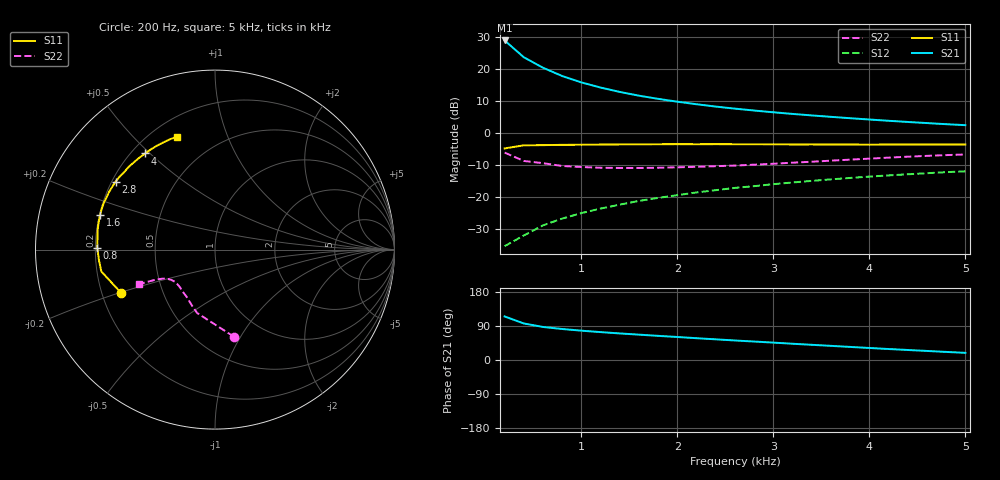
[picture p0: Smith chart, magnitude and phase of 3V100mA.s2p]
#  HZ  S  MA  R  50.0000
! Device:MCH4020
! Bias:VCE=3V, IC=100mA
!MHZ	S11(MAG/ANG)		S21(MAG/ANG)		S12(MAG/ANG)		S22(MAG/ANG)
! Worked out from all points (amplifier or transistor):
!   25 points, 200 Hz to 5 kHz, reference 50 ohm
!   highest |S21| = 29.0 dB at 200 Hz (marker M1)
!   |S21| within 3 dB of that: start of sweep to 314.1 Hz
!   unconditionally stable (mu >= 1): 1.61 kHz to 2.943 kHz
!   at 1 kHz: K = 0.96, MSG = 20.5 dB, |S12| = -25.0 dB
!   at 2.6 kHz: K = 1.00, MAG = 12.2 dB, |S12| = -17.1 dB
!   at 5 kHz: K = 0.94, MSG = 7.2 dB, |S12| = -11.9 dB
!   S11 on the Smith chart (normalised r, x): 200 Hz: 0.28, -0.20; 800 Hz: 0.21, +0.01; 1.6 kHz: 0.20, +0.14; 2.8 kHz: 0.21, +0.30; 4 kHz: 0.25, +0.48; 5 kHz: 0.30, +0.67
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200  0.577 -155.5  28.27 114.9  0.017 60.5  0.496 -77.8
400  0.645 -169.1  15.43 96.4  0.025 64.9  0.367 -105.8
600  0.649 -174.6  10.57 87.2  0.036 68.7  0.339 -111.9
800  0.656 179.3  7.841 81.8  0.046 70.5  0.306 -121.4
1000  0.658 174.4  6.227 77.4  0.056 71.3  0.295 -127.8
1200  0.663 170.4  5.172 73.6  0.066 71.6  0.287 -132.7
1400  0.666 166.8  4.421 70.1  0.076 71.2  0.285 -136.0
1600  0.668 163.4  3.86 66.9  0.087 70.6  0.285 -138.9
1800  0.671 160.2  3.443 63.7  0.097 69.8  0.287 -141.5
2000  0.672 157.5  3.108 60.7  0.107 69.1  0.292 -143.6
2200  0.671 154.3  2.835 57.5  0.118 68.1  0.297 -145.5
2400  0.672 151.4  2.606 54.5  0.128 67.0  0.304 -147.0
2600  0.671 148.6  2.419 51.5  0.139 65.7  0.311 -148.5
2800  0.671 145.6  2.26 48.7  0.148 64.4  0.321 -149.6
3000  0.669 142.6  2.122 45.9  0.159 63.1  0.332 -150.9
3200  0.665 139.5  2.001 42.9  0.169 61.7  0.345 -151.7
3400  0.666 136.2  1.895 40.1  0.179 60.2  0.357 -152.5
3800  0.663 129.5  1.713 34.5  0.199 57.1  0.385 -153.6
4000  0.662 126.0  1.635 31.7  0.209 55.5  0.399 -154.0
4200  0.663 122.5  1.562 29.0  0.218 53.9  0.414 -154.4
4600  0.663 115.5  1.438 23.9  0.236 50.6  0.441 -155.0
5000  0.664 108.7  1.333 18.9  0.253 47.3  0.464 -155.7
